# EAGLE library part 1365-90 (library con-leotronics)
DUAL ROW STRAIGHT HEADER 1364 SERIES. 1.27mm x 1.27mm. Without Fixing Post. SMT Source: http://www.leotronics.co.uk/Conexcon/Data%20Sheets/sec.%20A/1364ing.pdf
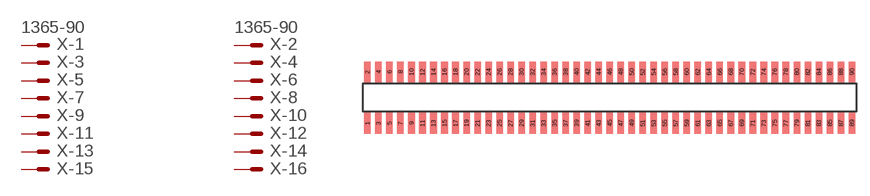
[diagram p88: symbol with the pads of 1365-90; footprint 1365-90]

Designator prefix X; gates -1=MVAL -2=MVAL -3=M -4=M -5=M -6=M -7=M -8=M -9=M -10=M -11=M -12=M -13=M -14=M -15=M -16=M -17=M -18=M -19=M -20=M -21=M -22=M -23=M -24=M -25=M -26=M -27=M -28=M -29=M -30=M -31=M -32=M -33=M -34=M -35=M -36=M -37=M -38=M -39=M -40=M -41=M -42=M -43=M -44=M -45=M -46=M -47=M -48=M -49=M -50=M -51=M -52=M -53=M -54=M -55=M -56=M -57=M -58=M -59=M -60=M -61=M -62=M -63=M -64=M -65=M -66=M -67=M -68=M -69=M -70=M -71=M -72=M -73=M -74=M -75=M -76=M -77=M -78=M -79=M -80=M -81=M -82=M -83=M -84=M -85=M -86=M -87=M -88=M -89=M -90=M

## 1365-90 (OC_FARNELL: unknown; OC_NEWARK: unknown)  [1365-90]
1  -1:S  pas
2  -2:S  pas
3  -3:S  pas
4  -4:S  pas
5  -5:S  pas
6  -6:S  pas
7  -7:S  pas
8  -8:S  pas
9  -9:S  pas
10  -10:S  pas
11  -11:S  pas
12  -12:S  pas
13  -13:S  pas
14  -14:S  pas
15  -15:S  pas
16  -16:S  pas
17  -17:S  pas
18  -18:S  pas
19  -19:S  pas
20  -20:S  pas
21  -21:S  pas
22  -22:S  pas
23  -23:S  pas
24  -24:S  pas
25  -25:S  pas
26  -26:S  pas
27  -27:S  pas
28  -28:S  pas
29  -29:S  pas
30  -30:S  pas
31  -31:S  pas
32  -32:S  pas
33  -33:S  pas
34  -34:S  pas
35  -35:S  pas
36  -36:S  pas
37  -37:S  pas
38  -38:S  pas
39  -39:S  pas
40  -40:S  pas
41  -41:S  pas
42  -42:S  pas
43  -43:S  pas
44  -44:S  pas
45  -45:S  pas
46  -46:S  pas
47  -47:S  pas
48  -48:S  pas
49  -49:S  pas
50  -50:S  pas
51  -51:S  pas
52  -52:S  pas
53  -53:S  pas
54  -54:S  pas
55  -55:S  pas
56  -56:S  pas
57  -57:S  pas
58  -58:S  pas
59  -59:S  pas
60  -60:S  pas
61  -61:S  pas
62  -62:S  pas
63  -63:S  pas
64  -64:S  pas
65  -65:S  pas
66  -66:S  pas
67  -67:S  pas
68  -68:S  pas
69  -69:S  pas
70  -70:S  pas
71  -71:S  pas
72  -72:S  pas
73  -73:S  pas
74  -74:S  pas
75  -75:S  pas
76  -76:S  pas
77  -77:S  pas
78  -78:S  pas
79  -79:S  pas
80  -80:S  pas
81  -81:S  pas
82  -82:S  pas
83  -83:S  pas
84  -84:S  pas
85  -85:S  pas
86  -86:S  pas
87  -87:S  pas
88  -88:S  pas
89  -89:S  pas
90  -90:S  pas

## Footprint 1365-90 (pad centres in mm)
DUAL ROW STRAIGHT HEADER 1364 SERIES. 1.27mm x 1.27mm. Without Fixing Post. SMT Source: http://www.leotronics.co.uk/Conexcon/Data%20Sheets/sec.%20A/1364ing.pdf
smd 0.76 x 2.4: 1 -27.94,-2.95; 2 -27.94,2.95; 3 -26.67,-2.95; 4 -26.67,2.95; 5 -25.4,-2.95; 6 -25.4,2.95; 7 -24.13,-2.95; 8 -24.13,2.95; 9 -22.86,-2.95; 10 -22.86,2.95; 11 -21.59,-2.95; 12 -21.59,2.95; 13 -20.32,-2.95; 14 -20.32,2.95; 15 -19.05,-2.95; 16 -19.05,2.95; 17 -17.78,-2.95; 18 -17.78,2.95; 19 -16.51,-2.95; 20 -16.51,2.95; 21 -15.24,-2.95; 22 -15.24,2.95; 23 -13.97,-2.95; 24 -13.97,2.95; 25 -12.7,-2.95; 26 -12.7,2.95; 27 -11.43,-2.95; 28 -11.43,2.95; 29 -10.16,-2.95; 30 -10.16,2.95; 31 -8.89,-2.95; 32 -8.89,2.95; 33 -7.62,-2.95; 34 -7.62,2.95; 35 -6.35,-2.95; 36 -6.35,2.95; 37 -5.08,-2.95; 38 -5.08,2.95; 39 -3.81,-2.95; 40 -3.81,2.95; 41 -2.54,-2.95; 42 -2.54,2.95; 43 -1.27,-2.95; 44 -1.27,2.95; 45 0,-2.95; 46 0,2.95; 47 1.27,-2.95; 48 1.27,2.95; 49 2.54,-2.95; 50 2.54,2.95; 51 3.81,-2.95; 52 3.81,2.95; 53 5.08,-2.95; 54 5.08,2.95; 55 6.35,-2.95; 56 6.35,2.95; 57 7.62,-2.95; 58 7.62,2.95; 59 8.89,-2.95; 60 8.89,2.95; 61 10.16,-2.95; 62 10.16,2.95; 63 11.43,-2.95; 64 11.43,2.95; 65 12.7,-2.95; 66 12.7,2.95; 67 13.97,-2.95; 68 13.97,2.95; 69 15.24,-2.95; 70 15.24,2.95; 71 16.51,-2.95; 72 16.51,2.95; 73 17.78,-2.95; 74 17.78,2.95; 75 19.05,-2.95; 76 19.05,2.95; 77 20.32,-2.95; 78 20.32,2.95; 79 21.59,-2.95; 80 21.59,2.95; 81 22.86,-2.95; 82 22.86,2.95; 83 24.13,-2.95; 84 24.13,2.95; 85 25.4,-2.95; 86 25.4,2.95; 87 26.67,-2.95; 88 26.67,2.95; 89 27.94,-2.95; 90 27.94,2.95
